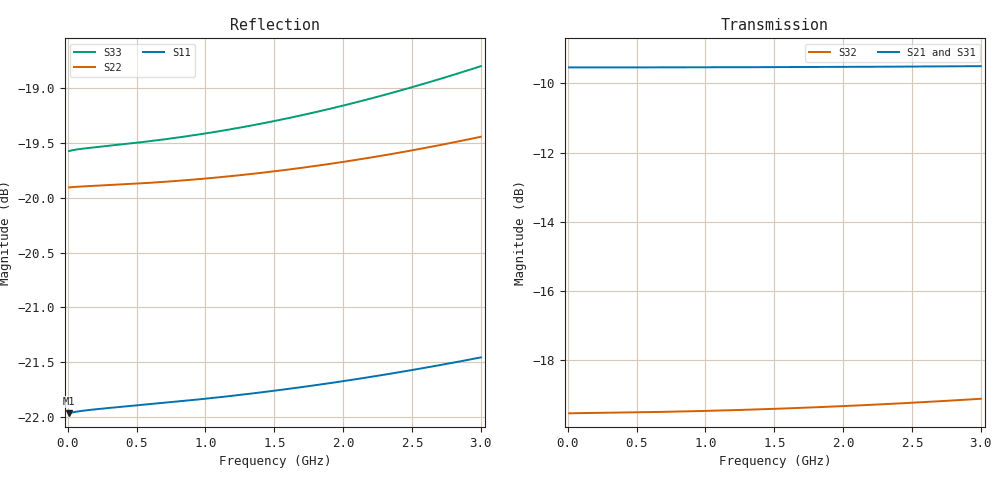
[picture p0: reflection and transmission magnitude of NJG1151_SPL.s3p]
! Created Fri Aug 03 15:49:09 2012
# hz S ma R 50
! 3 Port Network Data Splitter section Port1:SPLIN  Port2:SPLOUT1  Port3:SPLOUT2
! freq  magS11  angS11  magS12  angS12  magS13  angS13
!  magS21  angS21
!  magS22  angS22  magS23  angS23
!  magS31  angS31  magS32  angS32
!  magS33  angS33
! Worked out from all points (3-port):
!   300 points, 10 MHz to 3 GHz, reference 50 ohm
!   strongest paths, dB at 10 MHz, 760 MHz, 1.51 GHz, 2.26 GHz, 3 GHz:
!     S21: -9.5, -9.5, -9.5, -9.5, -9.5
!     S31: -9.6, -9.6, -9.6, -9.6, -9.6
!     S32: -19.5, -19.5, -19.4, -19.3, -19.1
!   lowest |S11| = -22.0 dB at 10 MHz (marker M1), VSWR 1.17, Z = 58.7 + j0.0171 ohm
!   |S11| at or under -10 dB: start of sweep to end of sweep
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1e7  0.07974 0.1  0.3336 0.0  0.3319 -0.0
     0.3336 0.0  0.1011 0.1  0.1054 0.0
     0.3319 -0.0  0.1054 0.0  0.105 0.1
1.8e8  0.08005 1.0  0.3336 0.0  0.3318 -0.0
       0.3336 0.0  0.1013 0.8  0.1055 0.7
       0.3318 -0.0  0.1055 0.7  0.1054 1.2
5.7e8  0.08048 2.8  0.3336 0.2  0.3318 -0.1
       0.3336 0.2  0.1016 2.5  0.1058 2.1
       0.3318 -0.1  0.1058 2.1  0.1061 3.5
8.8e8  0.08083 4.2  0.3337 0.2  0.3318 -0.2
       0.3337 0.2  0.1019 3.8  0.1061 3.3
       0.3318 -0.2  0.1061 3.3  0.1067 5.3
1.2e9  0.08123 5.5  0.3338 0.3  0.3318 -0.2
       0.3338 0.3  0.1023 5.2  0.1065 4.4
       0.3318 -0.2  0.1065 4.4  0.1075 7.0
1.51e9  0.08167 6.8  0.3339 0.4  0.3319 -0.3
        0.3339 0.4  0.1029 6.5  0.107 5.5
        0.3319 -0.3  0.107 5.5  0.1084 8.7
1.87e9  0.08225 8.3  0.3341 0.5  0.3321 -0.3
        0.3341 0.5  0.1036 7.9  0.1076 6.7
        0.3321 -0.3  0.1076 6.7  0.1097 10.6
2.24e9  0.08293 9.8  0.3343 0.6  0.3323 -0.4
        0.3343 0.6  0.1044 9.4  0.1085 8.0
        0.3323 -0.4  0.1085 8.0  0.1112 12.4
2.62e9  0.08371 11.3  0.3346 0.7  0.3325 -0.4
        0.3346 0.7  0.1055 10.9  0.1095 9.2
        0.3325 -0.4  0.1095 9.2  0.1129 14.3
3e9  0.08457 12.7  0.335 0.8  0.3328 -0.5
     0.335 0.8  0.1066 12.3  0.1106 10.4
     0.3328 -0.5  0.1106 10.4  0.1148 16.0
